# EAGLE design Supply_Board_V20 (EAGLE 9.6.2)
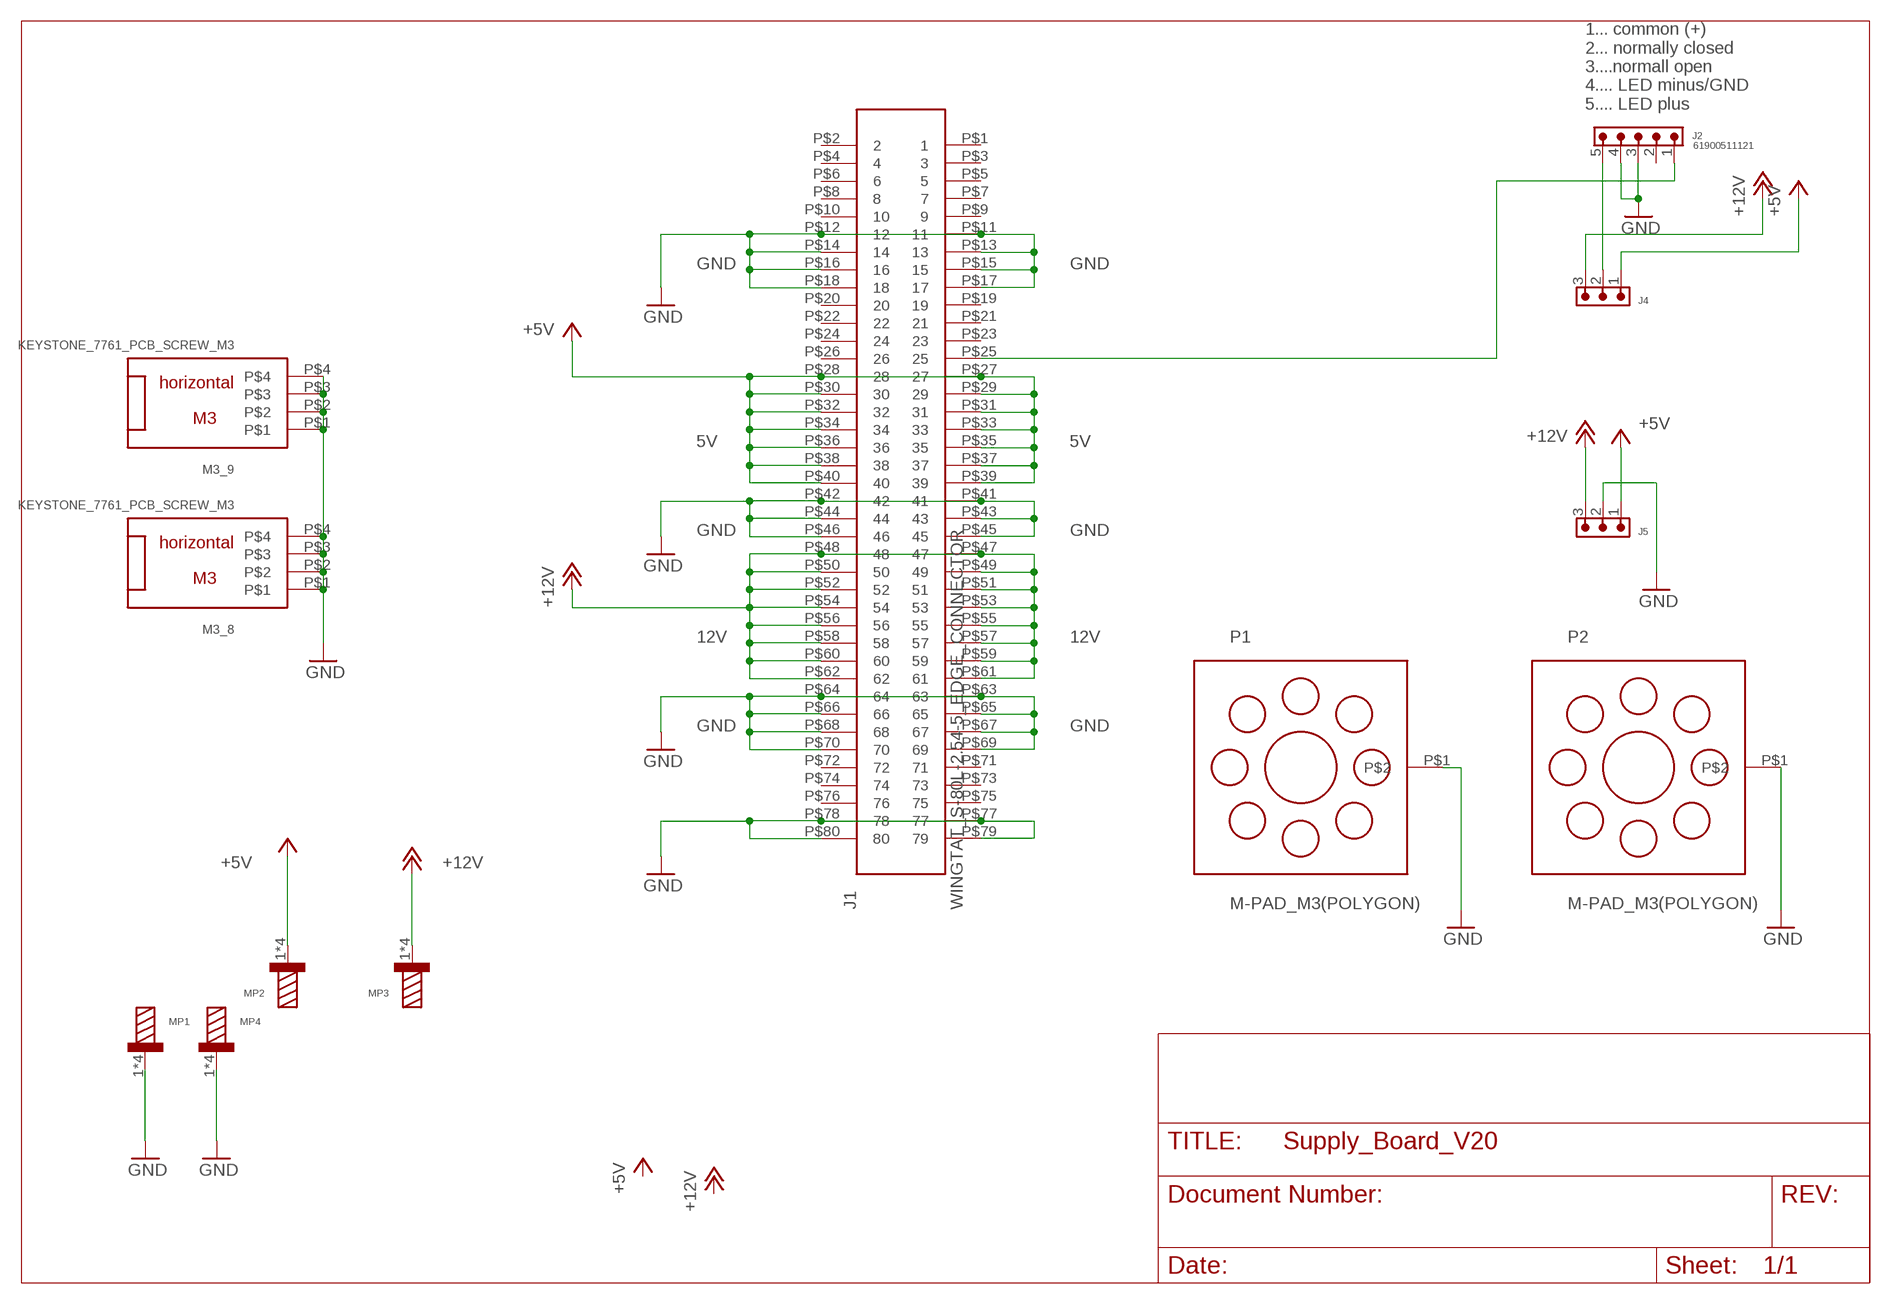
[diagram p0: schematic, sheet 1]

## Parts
J1  WINGTAT_S-80L-2.54-5_EDGE_CONNECTOR  [WINGTAT_S-80L-2.54-5_EDGE_CONNECTOR]
J2  61900511121  61900511121  [61900511121]
J4  6130XX11121_61300311121  [61300311121]
J5  6130XX11121_61300311121  [61300311121]
M3_8  KEYSTONE_7761_PCB_SCREW_M3  [KEYSTONE_7761_PCB_SCREW_M3]
M3_9  KEYSTONE_7761_PCB_SCREW_M3  [KEYSTONE_7761_PCB_SCREW_M3]
MP1  WP-THRSH_74651174R  [WP-THRSH_74651174]
MP2  WP-THRSH_74651174R  [WP-THRSH_74651174]
MP3  WP-THRSH_74651174R  [WP-THRSH_74651174]
MP4  WP-THRSH_74651174R  [WP-THRSH_74651174]
P1  M-PAD_M3(POLYGON)  [M-PAD_M3(POLYGON)]
P2  M-PAD_M3(POLYGON)  [M-PAD_M3(POLYGON)]

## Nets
+5V [Versorgung]: J1.P$27 J1.P$28 J1.P$29 J1.P$30 J1.P$31 J1.P$32 J1.P$33 J1.P$34 J1.P$35 J1.P$36 J1.P$37 J1.P$38 J1.P$39 J1.P$40 J4.1 J5.1 MP2.1 MP2.2 MP2.3 MP2.4
+12V [Versorgung]: J1.P$47 J1.P$48 J1.P$49 J1.P$50 J1.P$51 J1.P$52 J1.P$53 J1.P$54 J1.P$55 J1.P$56 J1.P$57 J1.P$58 J1.P$59 J1.P$60 J1.P$61 J1.P$62 J4.3 J5.3 MP3.1 MP3.2 MP3.3 MP3.4
GND [Versorgung]: J1.P$11 J1.P$12 J1.P$13 J1.P$14 J1.P$15 J1.P$16 J1.P$17 J1.P$18 J1.P$41 J1.P$42 J1.P$43 J1.P$44 J1.P$45 J1.P$46 J1.P$63 J1.P$64 J1.P$65 J1.P$66 J1.P$67 J1.P$68 J1.P$69 J1.P$70 J1.P$77 J1.P$78 J1.P$79 J1.P$80 J2.3 J2.4 J5.2 M3_8.P$1 M3_8.P$2 M3_8.P$3 M3_8.P$4 M3_9.P$1 M3_9.P$2 M3_9.P$3 M3_9.P$4 MP1.1 MP1.2 MP1.3 MP1.4 MP4.1 MP4.2 MP4.3 MP4.4 P1.P$1 P2.P$1
N$1: J2.5 J4.2
N$2: J1.P$25 J2.1
Unconnected: J1.P$1 J1.P$2 J1.P$3 J1.P$4 J1.P$5 J1.P$6 J1.P$7 J1.P$8 J1.P$9 J1.P$10 J1.P$19 J1.P$20 J1.P$21 J1.P$22 J1.P$23 J1.P$24 J1.P$26 J1.P$71 J1.P$72 J1.P$73 J1.P$74 J1.P$75 J1.P$76 J2.2

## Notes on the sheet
- 1... common (+)
  2... normally closed
  3....normall open
  4.... LED minus/GND
  5.... LED plus
- GND | GND
- 5V | 5V
- GND | GND
- 12V | 12V
- GND | GND

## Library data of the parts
J1 = Antec-Hood:WINGTAT_S-80L-2.54-5_EDGE_CONNECTOR
J2 = Eagle_WR-WTB (rev20a):61900511121: WR-WTB 2.54 mm Male Locking Header KIND PROPERTIES: Pitch:2.54 mm Gender:Male MATERIAL PROPERTIES: Insulator Material :PA66 Insulator Flammability Rating:UL94 V-0 Insulator Color:Beige Contact Material:Copper Alloy Contact Plating:Tin Contact Type:Stamped GENERAL INFORMATION Operating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; CONTACT-RESISTANCE: 20mOhm; DATASHEET-URL: https://www.we-online.com/catalog/datasheet/61900511121.pdf; GENDER: Male; L: 12.7mm; MOUNT: THT; PACKAGING: Bag; PART-NUMBER: 61900511121; PCB-CABLE-PANEL: PCB; PINS: 5; PITCH: 2.54mm; TOL-R: max.; TYPE: Vertical; USE-WITH: WR-WTB 2.54 mm Female Terminal Housing; WORKING-VOLTAGE: 250V(AC)
J4 J5 = Eagle_WR-PHD (rev19a):6130XX11121_61300311121: WR-PHD 2.54 mm THT Pin Header ARTICLE PROPERTIES: Pins:1;​ 2;​ 3;​ 4;​ 5;​ 6;​ 7;​ 8;​ 9;​ 10;​ 12;​ 13;​ 14;​ 15;​ 16;​ 18;​ 20;​ 22;​ 24;​ 25;​ 32;​ 36;​ 40 KIND PROPERTIES: Pitch：2.54 mm Quality Class:3 as per CECC 75 301-802 Rows：Single Gender：Pin Header Type：Straight MATERIAL PROPERTIES: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; DATASHEET-URL: https://katalog.we-online.com/em/datasheet/61300311121.pdf; GENDER: Pin Header; IR: 3A; MATES: WR-PHD 2.54mm Angled Socket Header /SMT Socket Header/Socket Header; PACKAGING: Bag; PART-NUMBER: 61300311121; PINS: 3; ROWS: Single; TYPE: Straight
M3_8 M3_9 = Antec-Hood:KEYSTONE_7761_PCB_SCREW_M3: Keystone_7761_PCB_Screw_M3_horizontal_15A
MP1-MP4 = Eagle_WP-THRSH (rev19a):WP-THRSH: WP-THRSH REDCUBE THR with external thread; DATASHEET-URL: https://katalog.we-online.de/em/datasheet/74651174R.pdf; IR: 50A; PART-NUMBER: 74651174R; PINS: 4; THREAD: M4
P1 P2 = Antec-Hood:M-PAD_M3(POLYGON)

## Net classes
1 Versorgung: width 1 mm, drill 1 mm, clearance 1 mm

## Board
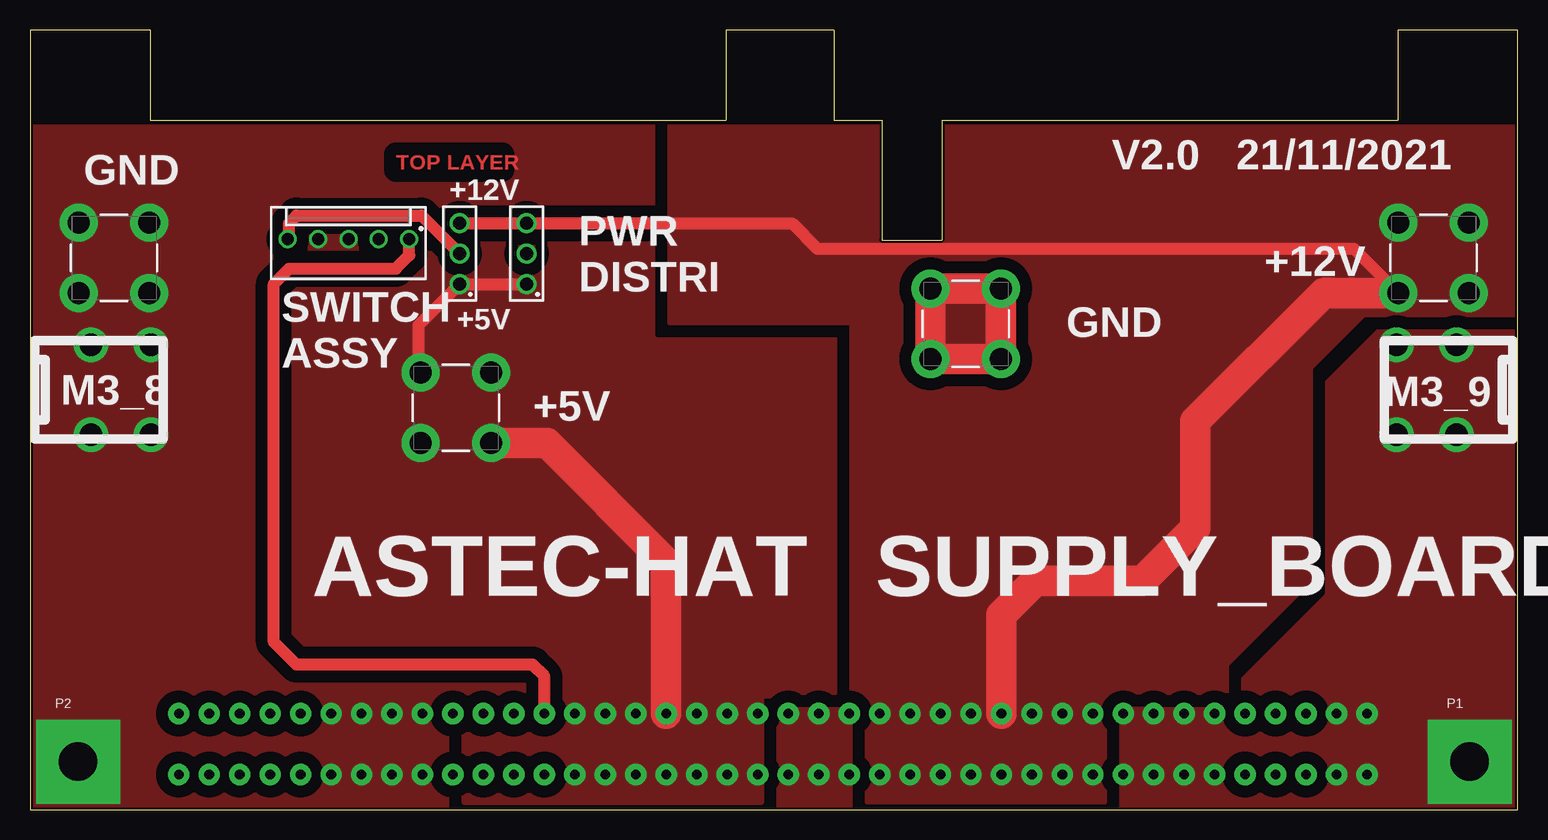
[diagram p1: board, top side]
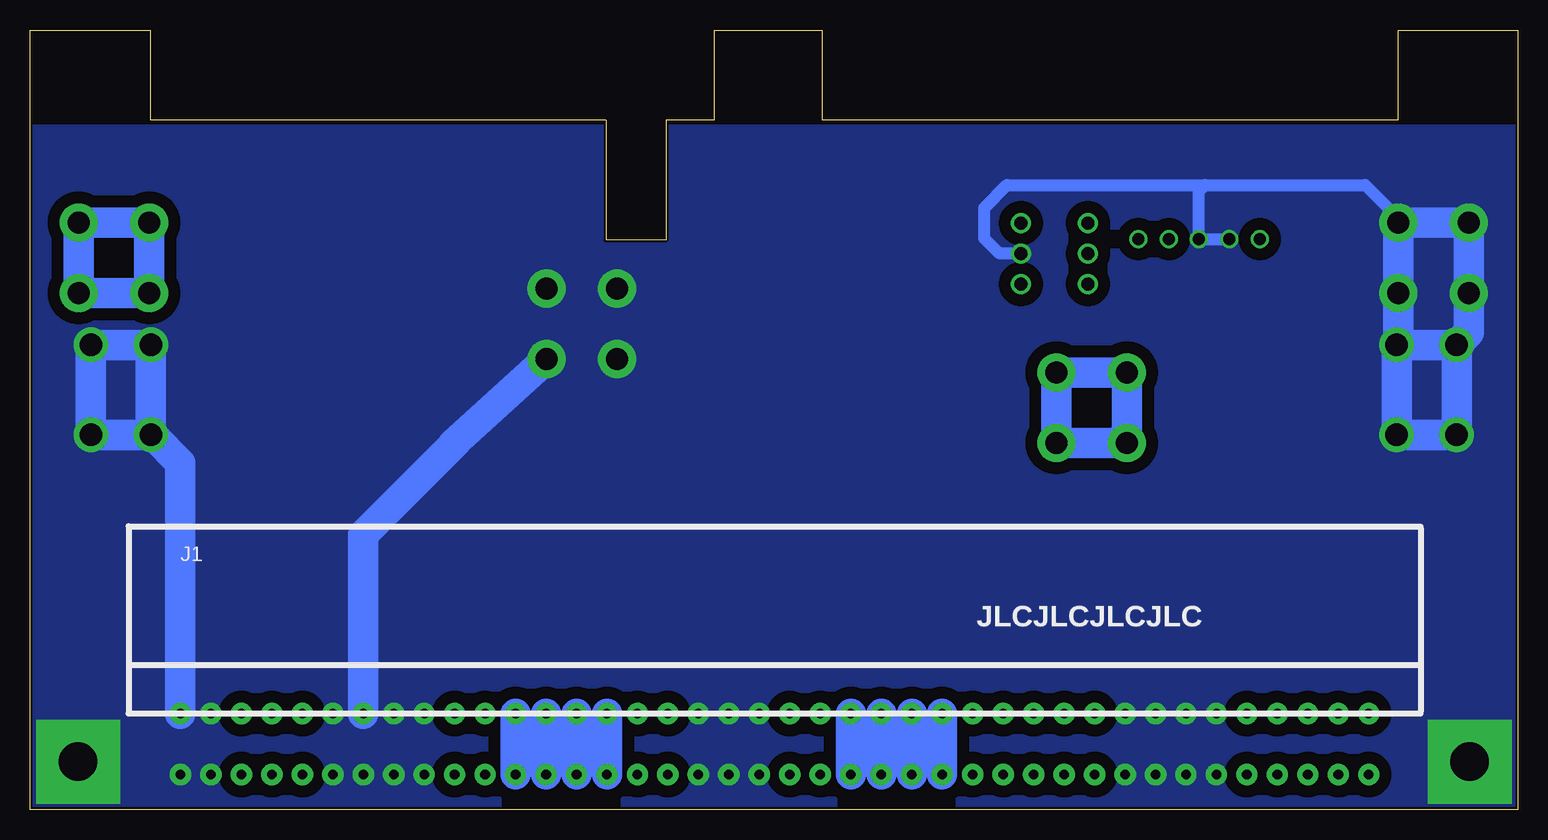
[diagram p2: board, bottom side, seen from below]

Size 124 x 65 mm. Coordinates in mm from the lower left corner, seen from the top.
Outline: 0,0 124,0 124,65 114,65 114,57.5 76,57.5 76,47.5 71,47.5 71,57.5 67,57.5 67,65 58,65 58,57.5 10,57.5 10,65 0,65 0,0
Copper layers (1*16): Top 0.035mm / dielectric 1.5mm / Bottom 0.035mm
Design rules "JLCPCB_2alyer": minimum track width 5mil, minimum drill 0.2mm, track to track 5mil, track to pad 0.2mm, pad to pad 0.2mm, via to via 0.2mm, smd to smd 5mil, copper to edge 0.2mm, drill to drill 0.5mm, minimum pad ring 0.13mm, minimum via ring 0.13mm, stop-mask expansion 0.05mm, vias tented up to drill 0mil, thermal gap 10mil
tRestrict: area 0,57.2 to 124.5,65.4
bRestrict: area 0,57.2 to 124.5,65.4; area 0,57.2 to 124.5,65.4; area 0,57.2 to 124.5,65.4; area 0,57.2 to 124.5,65.4; area 0,57.2 to 124.5,65.4

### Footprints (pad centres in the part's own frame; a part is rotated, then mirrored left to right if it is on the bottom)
WINGTAT_S-80L-2.54-5_EDGE_CONNECTOR = drill 0.8 pad 1.778: P$1 0,0; P$2 0,-5.08; P$3 -2.54,0; P$4 -2.54,-5.08; P$5 -5.08,0; P$6 -5.08,-5.08; P$7 -7.62,0; P$8 -7.62,-5.08; P$9 -10.16,0; P$10 -10.16,-5.08; P$11 -12.7,0; P$12 -12.7,-5.08; P$13 -15.24,0; P$14 -15.24,-5.08; P$15 -17.78,0; P$16 -17.78,-5.08; P$17 -20.32,0; P$18 -20.32,-5.08; P$19 -22.86,0; P$20 -22.86,-5.08; P$21 -25.4,0; P$22 -25.4,-5.08; P$23 -27.94,0; P$24 -27.94,-5.08; P$25 -30.48,0; P$26 -30.48,-5.08; P$27 -33.02,0; P$28 -33.02,-5.08; P$29 -35.56,0; P$30 -35.56,-5.08; P$31 -38.1,0; P$32 -38.1,-5.08; P$33 -40.64,0; P$34 -40.64,-5.08; P$35 -43.18,0; P$36 -43.18,-5.08; P$37 -45.72,0; P$38 -45.72,-5.08; P$39 -48.26,0; P$40 -48.26,-5.08; P$41 -50.8,0; P$42 -50.8,-5.08; P$43 -53.34,0; P$44 -53.34,-5.08; P$45 -55.88,0; P$46 -55.88,-5.08; P$47 -58.42,0; P$48 -58.42,-5.08; P$49 -60.96,0; P$50 -60.96,-5.08; P$51 -63.5,0; P$52 -63.5,-5.08; P$53 -66.04,0; P$54 -66.04,-5.08; P$55 -68.58,0; P$56 -68.58,-5.08; P$57 -71.12,0; P$58 -71.12,-5.08; P$59 -73.66,0; P$60 -73.66,-5.08; P$61 -76.2,0; P$62 -76.2,-5.08; P$63 -78.74,0; P$64 -78.74,-5.08; P$65 -81.28,0; P$66 -81.28,-5.08; P$67 -83.82,0; P$68 -83.82,-5.08; P$69 -86.36,0; P$70 -86.36,-5.08; P$71 -88.9,0; P$72 -88.9,-5.08; P$73 -91.44,0; P$74 -91.44,-5.08; P$75 -93.98,0; P$76 -93.98,-5.08; P$77 -96.52,0; P$78 -96.52,-5.08; P$79 -99.06,0; P$80 -99.06,-5.08
61900511121 = drill 1: 1 5.08,0.3; 2 2.54,0.3; 3 0,0.3; 4 -2.54,0.3; 5 -5.08,0.3
61300311121 = drill 1.1: 1 -2.54,0; 2 0,0; 3 2.54,0
KEYSTONE_7761_PCB_SCREW_M3 = drill 1.9: P$1 5.08,-3.75; P$2 5.08,3.75; P$3 10.08,3.75; P$4 10.08,-3.75
WP-THRSH_74651174 = drill 1.85 pad 3.2: 1 -2.935,-2.935; 2 -2.935,2.935; 3 2.935,2.935; 4 2.935,-2.935
M-PAD_M3(POLYGON) = drill 3.2 pad 7 square: P$1 0,0

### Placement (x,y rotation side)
J1  12.4,8 0 bottom
J2  26.54,47.24 0 top
J4  35.81,46.35 90 top
J5  41.4,46.35 90 top
M3_8  0,35 0 top
M3_9  124,35 180 top
MP1  7,46 0 top
MP2  35.5,33.5 0 top
MP3  117,46 0 top
MP4  78,40.5 0 top
P1  120,4 0 top
P2  4,4 0 top

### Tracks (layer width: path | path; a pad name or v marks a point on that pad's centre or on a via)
+5V
  Top 1.016: J5.1 J4.1 32.38,40.39 32.38,36.62 MP2.2
  Top 2.54: MP2.4 43.09,30.57 53.04,20.62 J1.P$33
  Bottom 2.54: J1.P$35 J1.P$36 | J1.P$33 J1.P$34 | J1.P$31 J1.P$32 | J1.P$29 J1.P$30 | MP2.2 MP2.1 MP2.4 MP2.3 MP2.2
  pour Top (rank 2, no thermals): 67.31,9.53 67.31,57.15 66.04,58.42 20.32,58.42 19.05,57.15 19.05,12.06 20.95,10.16 33.66,10.16 36.2,7.62 36.2,0.64 60.96,0.64 60.96,9.53
+12V
  Top 1.016: J4.3 J5.3 63.5,48.9 65.65,46.75 110.38,46.75 MP3.1
  Top 2.54: MP3.1 107.83,43.06 97.16,32.38 97.16,23.5 92.71,19.05 83.82,19.05 80.98,16.21 J1.P$55
  Bottom 2.54: J1.P$57 J1.P$58 | J1.P$55 J1.P$56 | J1.P$53 J1.P$54 | J1.P$51 J1.P$52 | MP3.2 MP3.1 MP3.4 MP3.3 MP3.2
  pour Top: 53.34,61.59 53.34,40.64 80.01,40.64 80.64,41.27 80.64,60.33 80.01,60.96 79.38,61.59
  pour Top (no thermals): 68.58,9.53 68.58,58.42 69.22,59.05 123.83,59.05 125.09,57.78 125.09,41.27 111.12,41.27 106.68,36.83 106.68,19.05 99.69,12.06 99.69,9.53 89.53,9.53 89.53,0.64 69.85,0.64 69.85,9.53
GND
  Top 2.54: MP4.4 MP4.3 MP4.2 MP4.1 MP4.4
  Bottom 1.016: J5.2 43.18,46.35 44.45,47.62 44.45,50.16 42.55,52.07 26.04,52.07 | J2.4 J2.3 26.54,51.56 26.04,52.07 | 26.04,52.07 12.7,52.07 9.94,49.3 MP1.3
  Bottom 2: M3_9.P$3 113.78,31.11 113.67,31.11
  Bottom 2.54: M3_8.P$2 4.07,39.77 MP1.1 MP1.2 MP1.3 MP1.4 9.94,38.9 | 9.94,38.9 M3_8.P$3 M3_8.P$4 M3_8.P$1 M3_8.P$2 | M3_8.P$2 9.79,38.75 9.94,38.9 | J1.P$79 111.46,28.91 113.67,31.11 | J1.P$67 96.22,22.91 88.53,30.6 88.68,30.54 MP4.4 | M3_9.P$4 M3_9.P$1 M3_9.P$2 M3_9.P$3 M3_9.P$4
  pour Bottom (no thermals): -4.45,-3.17 -2.54,-5.08 125.73,-5.08 131.44,0.64 131.44,64.77 127,69.22 -3.17,69.22 -4.45,67.94 -4.45,63.5
  pour Top (rank 3, no thermals): -3.17,62.23 -3.17,-1.27 -1.27,-3.17 128.27,-3.17 128.91,-3.81 128.91,59.69 126.36,62.23
  pour Top (rank 3, no thermals): 0.64,14.61 0.64,0 0,-0.64 123.19,-0.64 124.46,0.64 124.46,18.41 123.83,19.05 5.08,19.05
N$1
  Top 1.016: J2.5 21.59,47.67 21.59,48.9 22.23,49.53 32.64,49.53 J4.2
N$2
  Top 1.016: J1.P$25 42.88,11.1 41.91,12.06 22.23,12.06 20.32,13.97 20.32,43.81 21.59,45.09 30.48,45.09 31.62,46.23 J2.1

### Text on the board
Top: TOP LAYER
tPlace: V2.0 21/11/2021 | GND | +12V | +12V | PWR / DISTRI | +5V | GND | SWITCH / ASSY | +5V | ASTEC-HAT | SUPPLY_BOARD
bPlace: JLCJLCJLCJLC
